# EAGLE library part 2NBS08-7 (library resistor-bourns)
BOURNS RESISTOR NETWORK
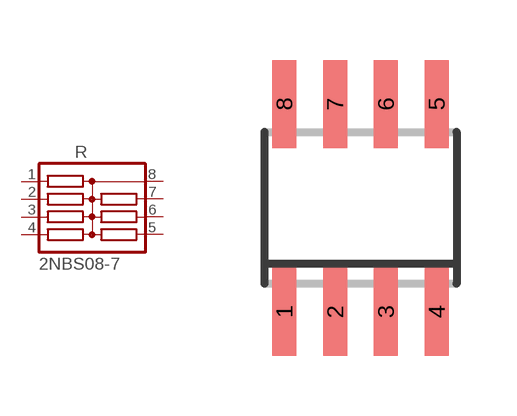
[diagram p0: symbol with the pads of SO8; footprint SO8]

Designator prefix R

## 2NBS08-7 (OC_FARNELL: unknown; OC_NEWARK: unknown)  [SO8]
1  1  pas
2  2  pas
3  3  pas
4  4  pas
5  5  pas
6  6  pas
7  7  pas
8  8  pas

## Footprint SO8 (pad centres in mm)
BOURNS RESISTOR NETWORK
smd 0.6 x 2.2: 1 -1.905,-2.6; 2 -0.635,-2.6; 3 0.635,-2.6; 4 1.905,-2.6; 5 1.905,2.6; 6 0.635,2.6; 7 -0.635,2.6; 8 -1.905,2.6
